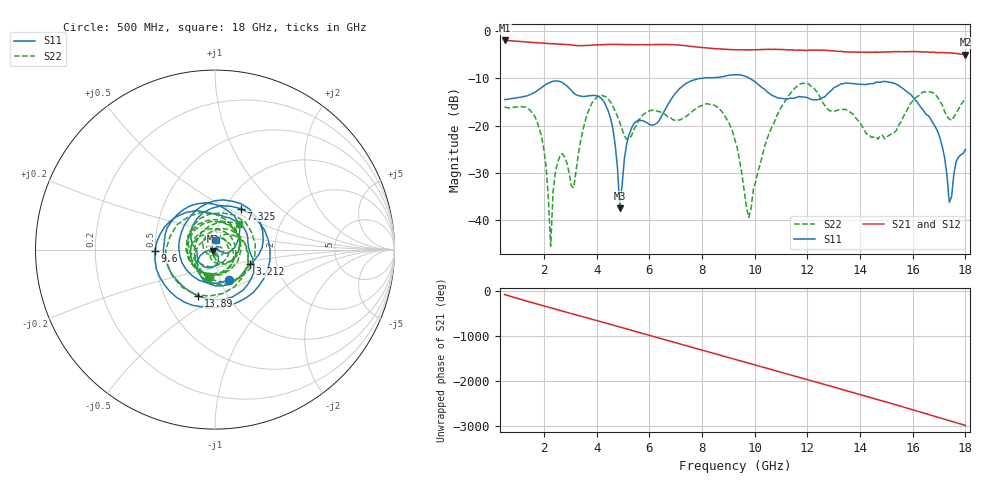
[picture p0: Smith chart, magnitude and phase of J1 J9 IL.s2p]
!Agilent Technologies,N5230A,MY45001360,A.07.50.67
!Agilent N5230A: A.07.50.67
!Date: Tuesday, April 16, 2024 16:39:54
!Correction: S11(Full 2 Port(1,2))
!S21(Full 2 Port(1,2))
!S12(Full 2 Port(1,2))
!S22(Full 2 Port(1,2))
!S2P File: Measurements: S11, S21, S12, S22:
# Hz S  dB  R 50
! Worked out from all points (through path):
!   201 points, 500 MHz to 18 GHz, reference 50 ohm
!   highest |S21| = -2.04 dB at 500 MHz (marker M1); lowest = -5.0 dB at 18 GHz (marker M2)
!   group delay of S21, straight-line fit = 459 ps
!   lowest |S11| = -37.4 dB at 4.875 GHz (marker M3), VSWR 1.03, Z = 49 - j0.869 ohm
!   |S11| at or under -10 dB: start of sweep to 8.017 GHz; 9.787 GHz to end of sweep
!   |S22| runs from -45.5 to -11.0 dB; largest |S21 - S12| = 0.0082
!   S11 on the Smith chart (normalised r, x): 500 MHz: 1.10, -0.39; 3.212 GHz: 1.46, -0.25; 7.325 GHz: 1.18, +0.58; 9.6 GHz: 0.50, -0.01; 13.89 GHz: 0.73, -0.41; 18 GHz: 1.01, +0.11
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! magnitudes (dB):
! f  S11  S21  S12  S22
! 500 MHz  -14.5  -2.0  -2.0  -16.1
! 1.725 GHz  -12.7  -2.5  -2.5  -19.0
! 2.075 GHz  -11.3  -2.7  -2.6  -28.7
! 2.25 GHz  -10.9  -2.7  -2.7  -45.5
! 2.513 GHz  -10.6  -2.8  -2.8  -27.8
! 3.212 GHz  -13.5  -3.1  -3.1  -29.5
! 3.475 GHz  -13.9  -3.1  -3.1  -20.9
! 4.438 GHz  -17.0  -2.9  -2.9  -14.5
! 4.875 GHz  -37.4  -2.9  -2.9  -19.4
! 5.312 GHz  -20.7  -2.9  -2.9  -22.2
! 6.362 GHz  -19.0  -2.9  -2.9  -17.0
! 7.325 GHz  -11.4  -3.1  -3.1  -18.4
! 9.25 GHz  -9.3  -4.0  -4.0  -23.0
! 9.6 GHz  -9.5  -4.0  -4.1  -33.9
! 9.775 GHz  -10.0  -4.0  -4.0  -39.4
! 11 GHz  -14.2  -4.0  -3.9  -16.1
! 12.22 GHz  -14.6  -4.1  -4.1  -11.9
! 13.89 GHz  -11.2  -4.5  -4.5  -18.7
! 15.11 GHz  -10.8  -4.5  -4.4  -22.0
! 16.95 GHz  -21.3  -4.6  -4.6  -14.1
! 17.39 GHz  -36.2  -4.7  -4.7  -18.6
! 18 GHz  -25.0  -5.0  -5.0  -14.1
